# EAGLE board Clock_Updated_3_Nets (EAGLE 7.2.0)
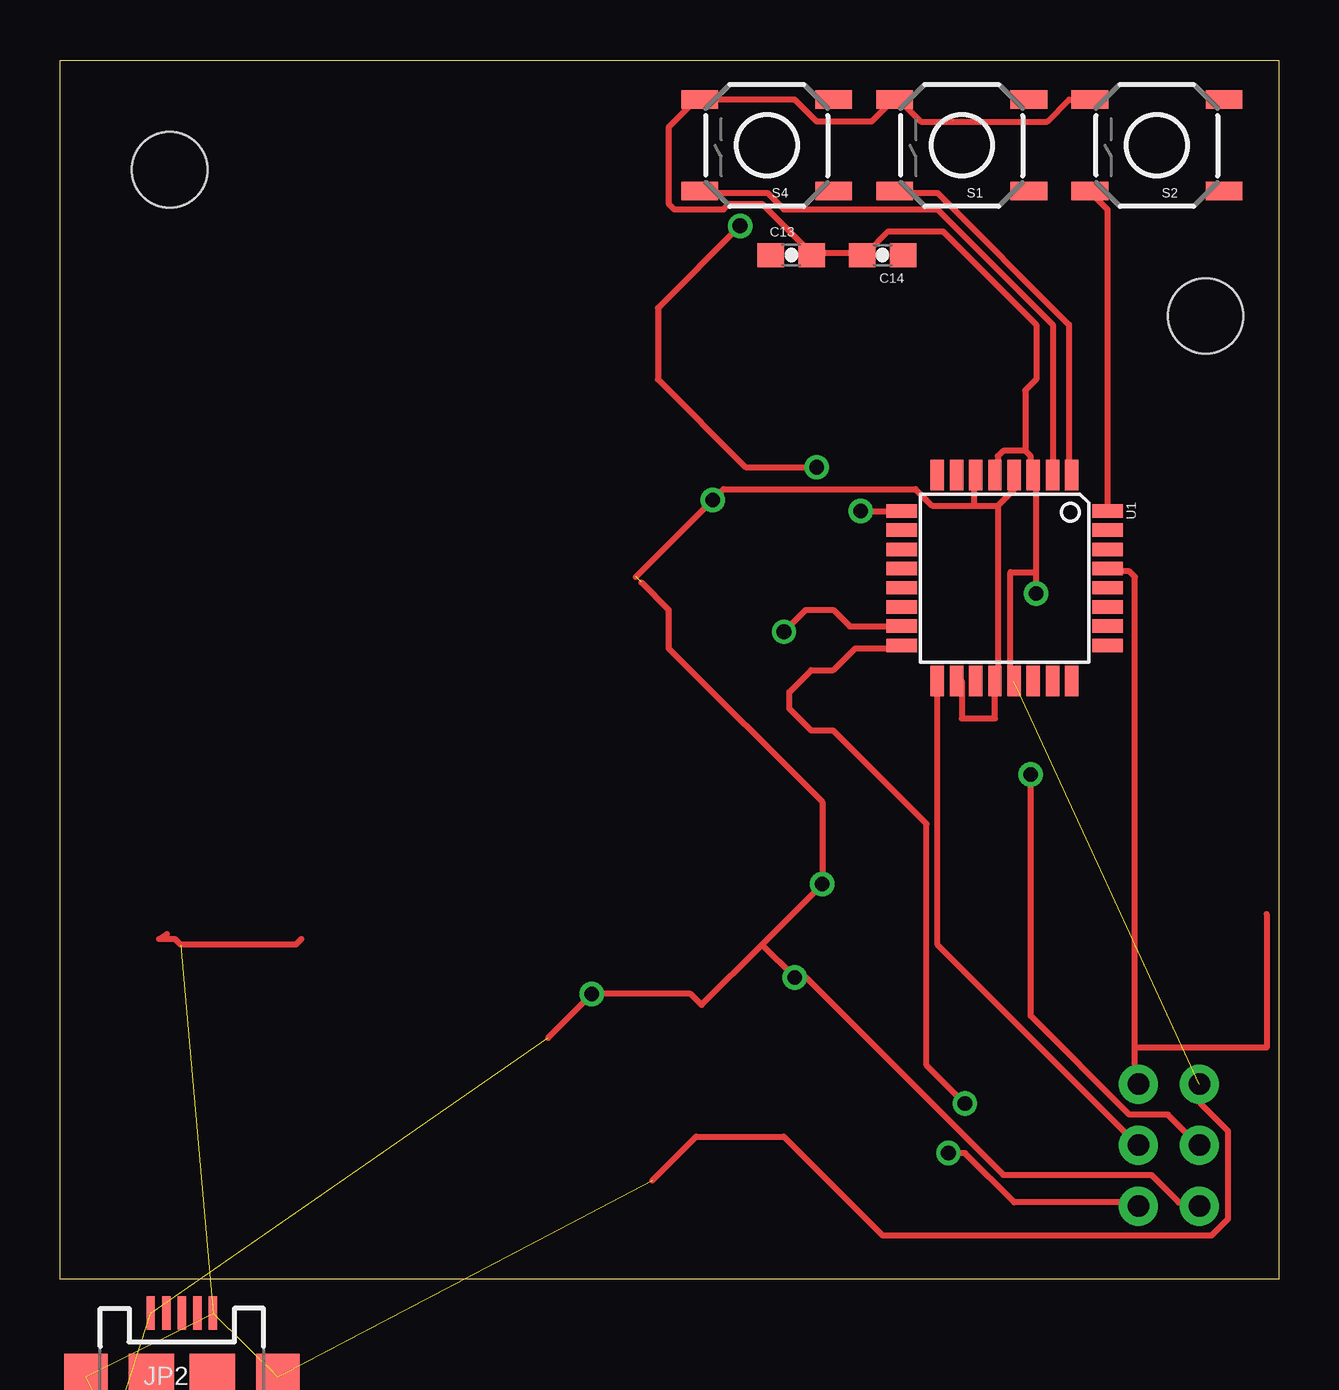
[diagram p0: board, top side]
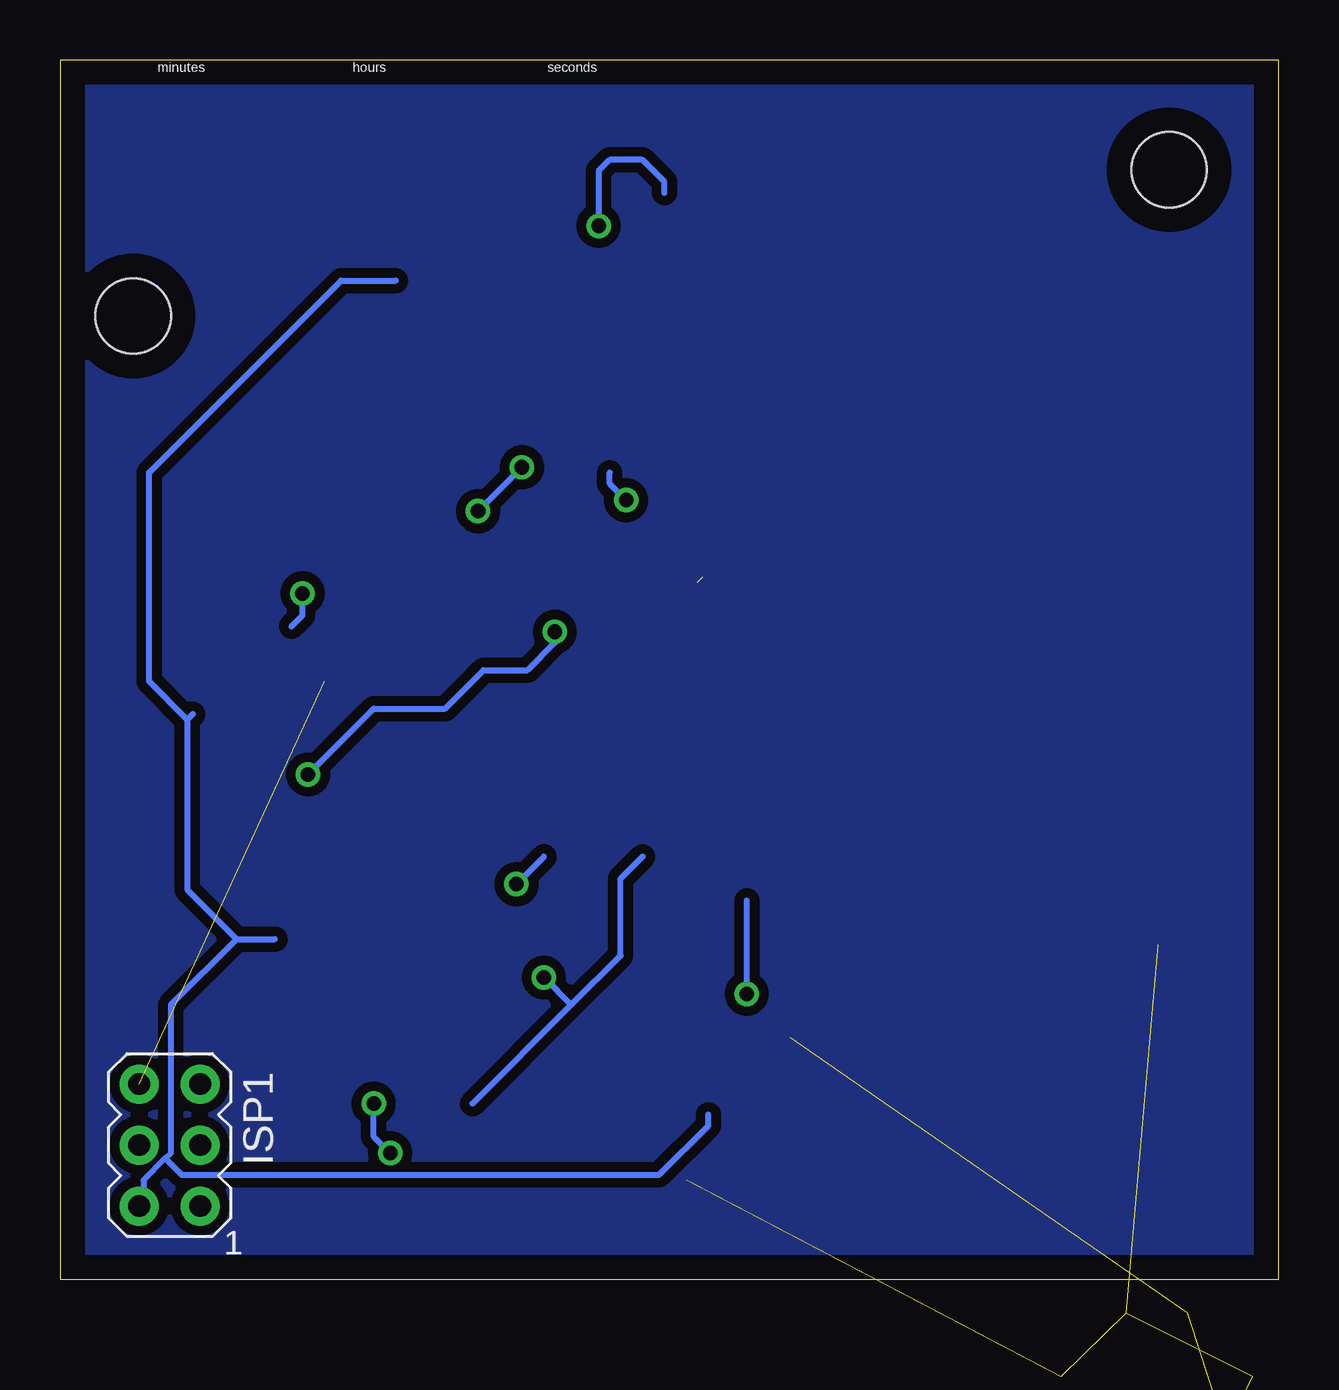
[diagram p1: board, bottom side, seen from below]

Size 50.8 x 50.8 mm. Coordinates in mm from the lower left corner, seen from the top.
Outline: 50.8,0 0,0 0,50.8 50.8,50.8 50.8,0
Copper layers (1*16): Top 0.035mm / dielectric 1.5mm / Bottom 0.035mm
Design rules "default": minimum track width 10mil, minimum drill 24mil, track to track 8mil, track to pad 8mil, pad to pad 8mil, via to via 8mil, smd to smd 8mil, copper to edge 40mil, drill to drill 8mil, minimum pad ring 10mil, minimum via ring 8mil, stop-mask expansion 4mil, vias tented up to drill 0mil, thermal gap 10mil
Holes 3.14 mm at 4.57,46.23 47.75,40.13

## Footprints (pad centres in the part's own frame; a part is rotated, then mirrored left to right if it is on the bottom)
0603-CAP = smd 1.1 x 1: 1 -0.85,0; 2 0.85,0
1206 = smd 1.6 x 1.8: 1 -1.4,0; 2 1.4,0
AVRISP = drill 0.9 pad 1.626: 1 -1.27,2.54; 2 1.27,2.54; 3 -1.27,0; 4 1.27,0; 5 -1.27,-2.54; 6 1.27,-2.54
USB-MICROB = smd 0.35 x 1.4: D+ 0,2.65; D- -0.65,2.65; GND 1.3,2.65; ID 0.65,2.65; VBUS -1.3,2.65 | smd 1.8 x 1.9: MT1 -4,0; MT2 4,0 | smd 1.9 x 1.9: P$1 -1.27,0; P$2 1.27,0
WS2812B = smd 1.5 x 0.9: 1-VDD 2.45,-1.65; 2-DOUT 2.45,1.65; 3-GND -2.45,1.65; 4-DIN -2.45,-1.65
TACTILE-SWITCH-SMD = smd 1.524 x 0.762: 1 -2.794,1.905; 2 2.794,1.905; 3 -2.794,-1.905; 4 2.794,-1.905
TQFP32-08 = smd 1.27 x 0.559: 1 -4.293,2.8; 2 -4.293,2; 3 -4.293,1.2; 4 -4.293,0.4; 5 -4.293,-0.4; 6 -4.293,-1.2; 7 -4.293,-2; 8 -4.293,-2.8; 17 4.293,-2.8; 18 4.293,-2; 19 4.293,-1.2; 20 4.293,-0.4; 21 4.293,0.4; 22 4.293,1.2; 23 4.293,2; 24 4.293,2.8 | smd 0.559 x 1.27: 9 -2.8,-4.293; 10 -2,-4.293; 11 -1.2,-4.293; 12 -0.4,-4.293; 13 0.4,-4.293; 14 1.2,-4.293; 15 2,-4.293; 16 2.8,-4.293; 25 2.8,4.293; 26 2,4.293; 27 1.2,4.293; 28 0.4,4.293; 29 -0.4,4.293; 30 -1.2,4.293; 31 -2,4.293; 32 -2.8,4.293

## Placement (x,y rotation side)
C13  8pF  [0603-CAP]  30.48,42.67 0 top
C14  8pF  [0603-CAP]  34.29,42.67 180 top
C15  [1206]  not placed on the board
ISP1  AVRISP-6  [AVRISP]  46.23,5.59 180 bottom
JP2  USB-MICROB  [USB-MICROB]  5.08,-4.06 0 top
L1  WS2812B  [WS2812B]  not placed on the board
S1  TAC_SWITCHSMD  [TACTILE-SWITCH-SMD]  37.59,47.24 180 top
S2  TAC_SWITCHSMD  [TACTILE-SWITCH-SMD]  45.72,47.24 180 top
S4  TAC_SWITCHSMD  [TACTILE-SWITCH-SMD]  29.46,47.24 180 top
U1  ATMEGA328P  [TQFP32-08]  39.37,29.21 270 top

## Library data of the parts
C13 C14 = SparkFun-Capacitors; PROD_ID: CAP-07876
C15 = SparkFun-Passives
ISP1 L1 = adafruit
JP2 = SparkFun-Connectors; PROD_ID: CONN-09505
S1 S2 S4 = SparkFun-Electromechanical; PROD_ID: SWCH-08247
U1 = SparkFun-DigitalIC; PROD_ID: IC-09069

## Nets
GND: C13.2 C14.2 C15.2 ISP1.6 JP2.GND JP2.MT1 JP2.MT2 S1.4 S2.4 S4.4 U1.3 U1.5 U1.21
N$1: ISP1.4 U1.15
N$2: ISP1.1 U1.16
N$4: S2.2 U1.32
N$29: C14.1
N$30: S1.2 U1.1
N$34: ISP1.3 U1.17
N$36: ISP1.5 U1.29
N$37: S4.2 U1.2
N$43: U1.9
VCC: C15.1 ISP1.2 JP2.VBUS U1.4 U1.6 U1.18 U1.20

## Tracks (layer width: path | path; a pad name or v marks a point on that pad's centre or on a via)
GND  (via drill 0.61)  (6 unrouted)
  Top 0.254: 10.06,14.17 9.83,13.95 5.03,13.95 4.8,14.17 4.12,14.17 4.47,14.39 | 24.69,4.12 26.52,5.94 30.18,5.94 34.29,1.83 48.01,1.83 48.69,2.52 48.69,6.17 47.55,7.32 47.55,8 ISP1.6 | 40.23,34.52 39.32,34.52 39.09,34.29 39.09,33.6 U1.5 | 40.23,34.52 40.46,34.29 40.46,33.6 U1.3 40.69,33.38 40.69,29.46 | S2.4 42.06,49.15 41.15,48.23 35.89,48.23 34.98,49.15 S1.4 34.75,49.15 33.83,48.23 31.55,48.23 30.63,49.15 S4.4 26.52,49.15 25.38,48.01 25.38,44.81 25.6,44.58 27.66,44.58 27.89,44.81 29.26,44.81 31.32,42.75 C13.2 31.55,42.75 33.38,42.75 C14.2 33.6,42.75 34.52,43.66 36.8,43.66 40.69,39.78 40.69,37.49 40.23,37.03 40.23,34.52 | v40.69,28.57 40.69,29.46 | U1.21 39.62,24.92 39.62,29.46 40.69,29.46
  Bottom 0.254: v40.69,28.57 40.69,27.66 41.15,27.2
N$1  (via drill 0.61)
  Top 0.254: v30.18,26.98 31.09,27.89 32.23,27.89 32.92,27.2 34.98,27.2 U1.15 | v40.46,21.03 40.46,10.97 44.58,6.86 46.18,6.86 47.32,5.71 ISP1.4
  Bottom 0.254: v30.18,26.98 30.18,26.52 31.32,25.38 33.15,25.38 34.75,23.77 37.72,23.77 v40.46,21.03
N$2  (via drill 0.61)
  Top 0.254: v37.72,7.32 36.12,8.91 36.12,18.97 32.23,22.86 31.32,22.86 30.4,23.77 30.4,24.46 31.32,25.38 32.23,25.38 33.15,26.29 34.98,26.29 U1.16 | v37.03,5.26 37.72,5.26 39.78,3.2 44.81,3.2 ISP1.1
  Bottom 0.254: v37.72,7.32 37.72,5.94 v37.03,5.26
N$4
  Top 0.254: U1.32 43.66,44.58 42.98,45.26 S2.2
N$28
  pour Bottom (isolate 0.406): 0.51,50.29 50.29,50.29 50.8,50.29 50.8,0 0,0 0,50.29
N$30
  Top 0.254: U1.1 42.06,33.6 42.06,39.78 36.58,45.26 34.98,45.26 S1.2
N$34
  Top 0.254: U1.17 36.58,13.95 44.81,5.71 ISP1.3
N$36
  Top 0.254: 44.81,9.65 44.81,8.23 ISP1.5 | 44.81,9.65 44.81,29.26 44.58,29.49 43.66,29.49 U1.29 | 50.29,15.21 50.29,9.65 44.81,9.65
N$37
  Top 0.254: U1.2 41.38,33.6 41.38,39.78 36.58,44.58 30.18,44.58 29.49,45.26 26.75,45.26 S4.2
N$43  (via drill 0.61)
  Top 0.254: v33.38,32 34.98,32 U1.9 | v31.55,33.83 28.57,33.83 24.92,37.49 24.92,40.46 v28.35,43.89
  Bottom 0.254: v31.55,33.83 v33.38,32 | v28.35,43.89 28.35,46.18 27.89,46.63 26.52,46.63 25.6,45.72 25.6,45.26
VCC  (via drill 0.61)  (3 unrouted)
  Top 0.254: 20.34,10.06 v22.17,11.89 26.29,11.89 26.75,11.43 29.26,13.95 | 29.26,13.95 v31.77,16.46 31.77,19.89 25.38,26.29 25.38,27.89 24.23,29.03 | 29.26,13.95 v30.63,12.57 31.09,12.57 39.32,4.34 45.49,4.34 46.63,3.2 47.32,3.2 ISP1.2 | 39.09,32.23 39.09,24.92 U1.20 38.97,23.37 37.59,23.37 37.59,24.92 U1.18 | 39.09,32.23 39.78,32.92 39.78,33.38 U1.4 | 24,29.26 v27.2,32.46 27.66,32.92 35.66,32.92 36.35,32.23 38.1,32.23 | 38.1,32.23 39.09,32.23 | U1.6 38.1,33.5 38.1,32.23
  Bottom 0.254: 43.43,14.17 41.83,14.17 | 43.43,14.17 45.49,16.23 45.49,23.32 | 45.26,23.55 45.49,23.32 | 46.41,5.03 46.18,5.26 46.18,11.43 43.43,14.17 | 46.41,5.03 47.32,4.12 47.32,3.2 ISP1.2 | 23.77,6.86 23.77,6.4 25.83,4.34 45.72,4.34 46.41,5.03 | 26.52,17.6 27.43,16.69 27.43,13.49 29.49,11.43 | 33.6,7.32 29.49,11.43 | v22.17,11.89 22.17,15.77 | v31.77,16.46 30.63,17.6 | v30.63,12.57 29.49,11.43 | 27.89,33.6 27.89,33.15 v27.2,32.46 | 36.8,41.6 39.09,41.6 47.09,33.6 47.09,24.92 45.49,23.32

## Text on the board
bPlace: seconds | hours | minutes

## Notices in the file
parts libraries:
SparkFun-Capacitors: Licensing: Creative Commons ShareAlike 4.0 International - https://creativecommons.org/licenses/by-sa/4.0
